(* Logix 5000 DataType export Exlar_Status; software revision 32.02 *)

TYPE Exlar_Status :   // Tritex II Status
STRUCT
   EIP_Comm : INT;   // EIP module communication
   OutputEventsStatus : INT;   // 104
   OutputEventsMoveInPosition : INT;   // 108
   OutputEventsMotion : INT;   // 105
   OutputsEventsMotionActive : INT;   // 107
   PositionFeedback_low : INT;   // 378
   PositionFeedback_high : INT;
   SoftFaults : INT;   // 7
   HardFaults : INT;   // 6
   VelocityDisplay_low : INT;   // 356
   VelocityDisplay_high : INT;
   CurrentDisplay : INT;   // 567
   CurrentContinuous : INT;   // 565
   CurrentLimit : INT;   // 5108
   VoltageHallBattery : INT;   // 8
   VoltageBus : INT;   // 571
   TemperatureBoard : INT;   // 11
   TemperatureActuator : INT;   // 15
END_STRUCT
END_TYPE
